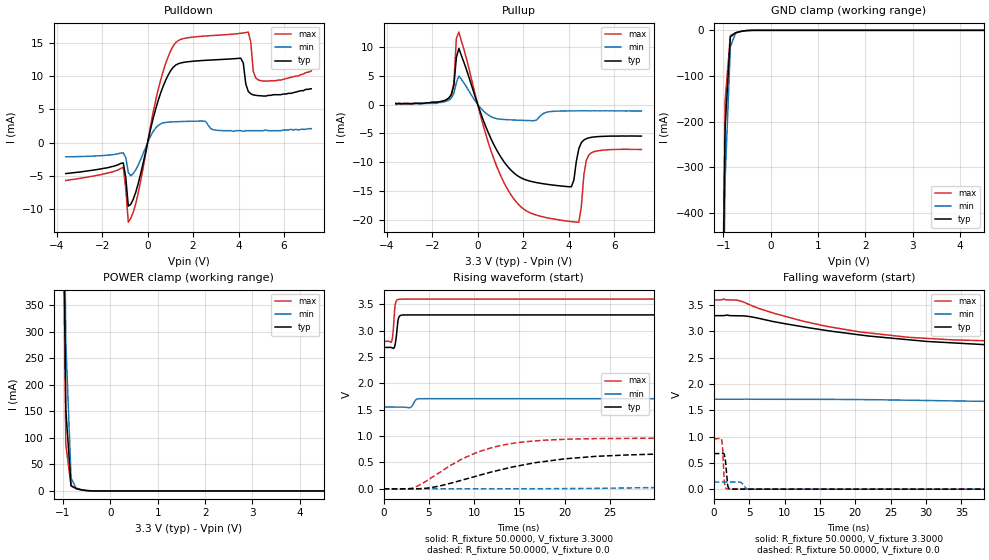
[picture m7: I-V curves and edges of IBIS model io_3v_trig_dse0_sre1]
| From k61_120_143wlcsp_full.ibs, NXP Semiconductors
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[Model]  io_3v_trig_dse0_sre1
|   Model io_3v_trig_dse0_sre1
| Library cells for typ/min/max conditions are connected as defined below:
|  pad - External Pad
|  ipp_do_3v - Core Input
|  ipp_obe_3v - Output Buffer Enable
|  esd_boost - vdd_s_3v
|  esd_trigger - vss_s_3v
|  ipp_ame_3v - vss_s_3v
|  ipp_dse_3v - vss_s_3v
|  ipp_ina_3v - NC
|  ipp_ina_mux_3v - NC
|  ipp_ind_3v - NC
|  ipp_pue_3v - vss_s_3v
|  ipp_sre_3v - vdd_s_3v
|  tie_3v - vdd_s_3v
|  tie_hi - vdd_s_lv
|  vbuf_3v - vdd_s_3v
|  vdd_s_3v - vdd_s_3v
|  vdd_s_lv - vdd_s_lv
|  vss_bulk - vss_s_3v
|  vss_s_3v - vss_s_3v
| All other pins connected to ground
Model_type I/O
Polarity   Non-Inverting
Enable   Active-High
Vinl =   1.1550V
Vinh =   2.3100V
Vmeas =  1.6500V
Cref =   25.0000pF
Rref =   50.0000
Vref =   0.0V
C_comp   1.9033pF   1.7921pF   2.1182pF
[Temperature Range]   25.0000   0.1250k   -40.0000
[Voltage Range]   3.3000V   1.7100V   3.6000V
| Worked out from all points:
|   slope of the pulldown table from 0 to 0.495 V, typ, clamps not added: 74.6 ohm
|   slope of the pullup table from 0 to 0.495 V, typ, clamps not added: 96.1 ohm
|   GND clamp passes 1 mA (typ) near -0.54 V on its own axis
|   POWER clamp passes 1 mA (typ) near -0.53 V on its own axis
|   rising waveform, R_fixture 50.0000, V_fixture 3.3000: 20-80 % time 230ps typ, 315ps min, 205ps max; typ from 2.68 V to 3.3 V
|   rising waveform, R_fixture 50.0000, V_fixture 0.0: 20-80 % time 10.8ns typ, 34ns min, 6.55ns max; typ from 0 V to 0.676 V
|   falling waveform, R_fixture 50.0000, V_fixture 3.3000: 20-80 % time 22ns typ, 52ns min, 16.6ns max; typ from 3.3 V to 2.68 V
|   falling waveform, R_fixture 50.0000, V_fixture 0.0: 20-80 % time 255ps typ, 472ps min, 215ps max; typ from 0.676 V to 0 V
[Pulldown]
|Voltage   I(typ)   I(min)   I(max)
-3.6V     -4.64mA    -2.13mA    -5.68mA
-1.07V    -3.05mA    -1.536mA   -3.686mA
-850mV    -9.531mA   -4.459mA   -11.94mA
-520mV    -7.433mA   -4.072mA   -9.157mA
580mV     7.512mA    2.843mA    9.473mA
1.46V     11.97mA    3.168mA    15.51mA
4.1V      12.68mA    1.8mA      16.42mA
4.43V     7.69mA     1.8mA      16.6mA
4.54V     7.33mA     1.8mA      15.1mA
4.65V     7.17mA     1.8mA      10.69mA
4.87V     7.06mA     1.8mA      9.41mA
7.2V      8.1mA      2.1mA      10.8mA
[Pullup]
|Voltage   I(typ)   I(min)   I(max)
-3.6V     200uA      0A         200uA
-1.27V    1.12mA     760uA      1.13mA
-1.05V    3.27mA     1.9mA      3.696mA
-940mV    8.16mA     3.801mA    11.47mA
-830mV    9.694mA    4.923mA    12.52mA
1.15V     -9.866mA   -2.586mA   -13.47mA
3.24V     -13.9mA    -1.205mA   -19.73mA
4.12V     -14.22mA   -1.1mA     -20.25mA
4.45V     -7.608mA   -1.09mA    -20.35mA
4.78V     -5.902mA   -1.09mA    -9.632mA
5V        -5.67mA    -1.1mA     -8.343mA
7.2V      -5.46mA    -1.11mA    -7.78mA
[GND_clamp]
|Voltage   I(typ)   I(min)   I(max)
-3.6V     -47.82A    -47.1A     -48.34A
-1.07V    -1.102A    -1.183A    -1.105A
-960mV    -210.7mA   -326mA     -154mA
-850mV    -14.47mA   -36.11mA   -11.11mA
-740mV    -5.262mA   -6.033mA   -5.843mA
-520mV    -636.9uA   -915.4uA   -467.5uA
-300mV    -2.578uA   -18.09uA   -370.9nA
7.2V      0A         0A         0A
[POWER_clamp]
|Voltage   I(typ)   I(min)   I(max)
-3.6V     36.98A     36.74A     37.19A
-1.05V    1.02A      1.161A     949.9mA
-940mV    152.3mA    280.6mA    87.35mA
-830mV    9.987mA    24.48mA    9.181mA
-720mV    4.227mA    4.408mA    5.116mA
-500mV    628.6uA    743.9uA    622.6uA
-390mV    66.57uA    164uA      29.9uA
7.2V      0A         0A         0A
[Ramp]
| variable   typ   min   max
dV/dt_r  0.4058/10.7521n   80.3144m/33.9644n   0.5758/6.5493n
dV/dt_f  0.3716/21.9741n   95.2446m/52.0567n   0.4822/16.5904n
R_load = 50.0000
[Rising Waveform]
R_fixture= 50.0000
V_fixture= 3.3000
V_fixture_min= 1.7100
V_fixture_max= 3.6000
|time   V(typ)   V(min)   V(max)
0s        2.681V     1.551V     2.796V
873.9ps   2.679V     1.551V     2.794V
1.053ns   2.665V     1.552V     2.991V
1.187ns   2.687V     1.552V     3.332V
1.337ns   2.801V     1.552V     3.54V
1.603ns   3.21V      1.552V     3.593V
1.889ns   3.292V     1.552V     3.598V
2.929ns   3.299V     1.541V     3.599V
4.276ns   3.299V     1.71V      3.599V
250ns     3.3V       1.71V      3.6V
[Rising Waveform]
R_fixture= 50.0000
V_fixture= 0.0
V_fixture_min= 0.0
V_fixture_max= 0.0
|time   V(typ)   V(min)   V(max)
0s        5.332nV    455.6nV    4.027nV
3.401ns   -65.29uV   -1.632mV   27.26mV
8.79ns    170.4mV    -17.84uV   576.4mV
11.64ns   306.7mV    26.09uV    765.9mV
15.55ns   456.4mV    541.1uV    891mV
20.44ns   574.6mV    4.018mV    942.2mV
29.58ns   655.3mV    21.43mV    958.1mV
44.29ns   674.9mV    62.41mV    959.5mV
87.36ns   676.3mV    126.3mV    959.6mV
250ns     676.3mV    133.9mV    959.6mV
[Falling Waveform]
R_fixture= 50.0000
V_fixture= 3.3000
V_fixture_min= 1.7100
V_fixture_max= 3.6000
|time   V(typ)   V(min)   V(max)
0s        3.3V       1.71V      3.6V
3.611ns   3.299V     1.71V      3.586V
7.282ns   3.221V     1.71V      3.398V
12.82ns   3.084V     1.71V      3.19V
20.67ns   2.934V     1.704V     2.991V
27.45ns   2.843V     1.693V     2.889V
39.99ns   2.737V     1.666V     2.817V
59.44ns   2.691V     1.624V     2.798V
113.2ns   2.681V     1.564V     2.796V
250ns     2.681V     1.551V     2.796V
[Falling Waveform]
R_fixture= 50.0000
V_fixture= 0.0
V_fixture_min= 0.0
V_fixture_max= 0.0
|time   V(typ)   V(min)   V(max)
0s        676.3mV    133.9mV    959.6mV
1.13ns    678mV      133.8mV    930.4mV
1.265ns   680.7mV    133.8mV    739.8mV
1.442ns   670.9mV    133.8mV    235.4mV
1.52ns    644.9mV    133.7mV    106.7mV
1.661ns   527.3mV    133.7mV    27.52mV
1.898ns   140.5mV    133.7mV    4.398mV
2.065ns   30.29mV    133.7mV    2.235mV
5.371ns   494.1uV    274.7uV    592.1uV
250ns     13.62nV    474.9nV    11.48nV
